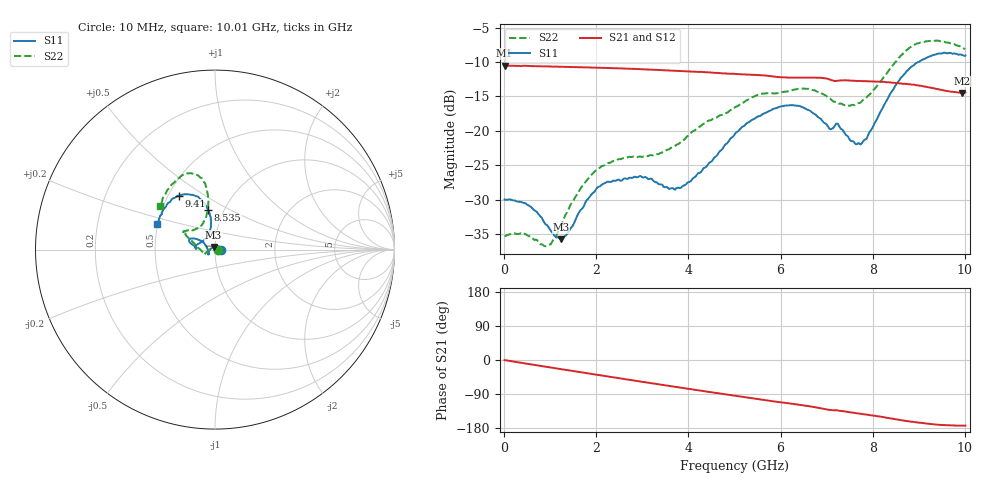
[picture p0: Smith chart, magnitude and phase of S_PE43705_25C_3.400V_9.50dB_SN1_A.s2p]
! Device ID: PE43705
! Serial: 1
! Insertion: A
! Impedance: 50 ohm
! Temp: 25C
! VDD: 3.400V
! Attenuation Step: 9.50dB
#  Hz  S  RI  R  50
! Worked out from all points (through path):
!   401 points, 10 MHz to 10.01 GHz, reference 50 ohm
!   highest |S21| = -10.52 dB at 10 MHz (marker M1); lowest = -14.5 dB at 9.935 GHz (marker M2)
!   group delay of S21, straight-line fit = 49.8 ps
!   lowest |S11| = -35.8 dB at 1.235 GHz (marker M3), VSWR 1.03, Z = 49.2 + j1.42 ohm
!   |S11| at or under -10 dB: start of sweep to 8.994 GHz
!   |S22| runs from -36.7 to -6.9 dB; largest |S21 - S12| = 0.0027
!   S11 on the Smith chart (normalised r, x): 10 MHz: 1.07, +0.00; 8.535 GHz: 0.84, +0.39; 9.41 GHz: 0.57, +0.39; 10.01 GHz: 0.50, +0.16
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1e7  0.0317 0.00014  0.2979 -0.00129  0.2983 -0.00128  0.0173 0.000279
5.1e8  0.0237 0.0166  0.2909 -0.0523  0.291 -0.0521  0.0109 0.0136
9.1e8  0.00766 0.0194  0.2795 -0.0905  0.2794 -0.0901  -0.00397 0.014
1.235e9  -0.00762 0.0144  0.2664 -0.1193  0.2665 -0.1189  -0.0192 0.00779
1.685e9  -0.0271 0.000579  0.2436 -0.1563  0.2436 -0.1562  -0.0389 -0.00557
2.21e9  -0.0383 -0.0176  0.2104 -0.1939  0.2105 -0.1938  -0.0535 -0.0206
2.935e9  -0.0388 -0.0262  0.1555 -0.2337  0.1558 -0.2336  -0.0618 -0.0204
3.36e9  -0.035 -0.0214  0.12 -0.249  0.1203 -0.2487  -0.0663 -0.0152
3.885e9  -0.0398 -0.000694  0.0749 -0.2608  0.0751 -0.2606  -0.0851 0.00247
5.01e9  -0.0804 0.0509  -0.0196 -0.258  -0.0193 -0.2581  -0.1377 0.0553
5.985e9  -0.137 0.0607  -0.0898 -0.2282  -0.0887 -0.2285  -0.1653 0.0914
6.685e9  -0.132 0.0319  -0.1339 -0.203  -0.1338 -0.2029  -0.1686 0.1032
7.06e9  -0.1028 0.0133  -0.1568 -0.1761  -0.1563 -0.1773  -0.1319 0.1101
7.335e9  -0.0976 0.0305  -0.1631 -0.1653  -0.1631 -0.1661  -0.1054 0.1162
7.71e9  -0.0538 0.0604  -0.18 -0.1438  -0.1795 -0.1439  -0.069 0.1436
7.91e9  -0.0342 0.0887  -0.1871 -0.1316  -0.1871 -0.1331  -0.0549 0.1728
8.36e9  -0.0241 0.1792  -0.2015 -0.1003  -0.2003 -0.1014  -0.0378 0.2757
8.535e9  -0.0395 0.22  -0.2044 -0.0861  -0.203 -0.0883  -0.044 0.3249
8.935e9  -0.0934 0.2945  -0.2072 -0.0581  -0.2062 -0.0566  -0.0979 0.4153
9.41e9  -0.2027 0.3008  -0.1987 -0.0321  -0.1975 -0.0316  -0.1847 0.4133
9.935e9  -0.3122 0.1713  -0.1872 -0.0226  -0.1885 -0.0229  -0.2937 0.2734
1.001e10  -0.3216 0.1436  -0.1885 -0.0229  -0.1889 -0.0236  -0.3065 0.2454
